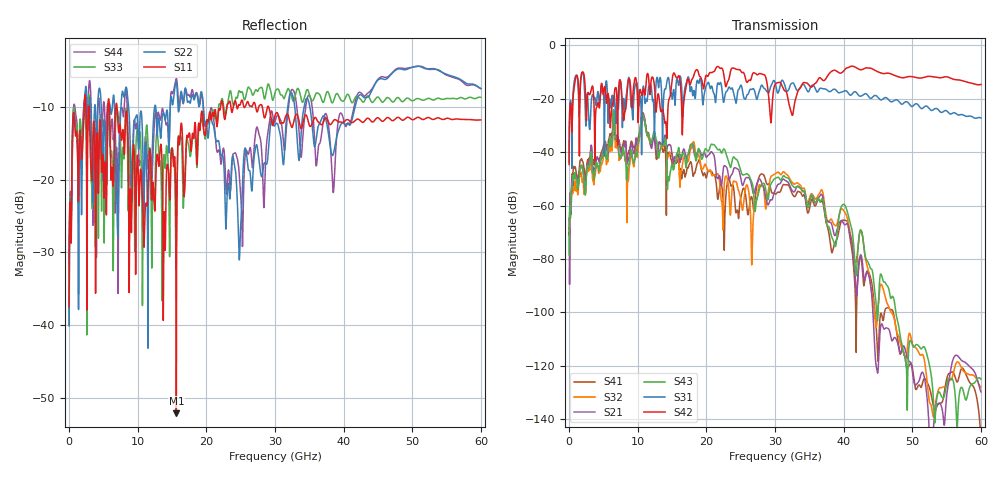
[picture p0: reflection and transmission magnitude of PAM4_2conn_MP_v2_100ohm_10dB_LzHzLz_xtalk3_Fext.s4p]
! Info: Touchstone file created by Circ.  Input file=FAB50GbE_2conn_Midplane_Examax_Topo2_v2_100ohm_10dB_LzHzLz.circ
# Hz S RI R 50
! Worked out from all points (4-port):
!   6000 points, 10 MHz to 60 GHz, reference 50 ohm
!   strongest paths, dB at 10 MHz, 15.01 GHz, 30.01 GHz, 45.01 GHz, 60 GHz:
!     S42: -44.7, -13.0, -14.7, -9.9, -14.7
!     S31: -43.6, -19.7, -13.9, -19.5, -27.2
!     S43: -78.4, -44.6, -49.9, -100.4, -125.0
!     S21: -64.7, -41.3, -54.3, -122.1, -129.7
!     S32: -69.2, -40.5, -48.2, -98.8, -128.0
!     S41: -68.5, -44.2, -55.6, -118.3, -146.4
!   lowest |S11| = -52.1 dB at 15.63 GHz (marker M1), VSWR 1.00, Z = 49.8 + j0.0187 ohm
!   |S11| at or under -10 dB: 2.897 GHz to 5.662 GHz (2.765 GHz wide, 64.6 % of centre); 6.985 GHz to 22.08 GHz (15.1 GHz wide, 104 % of centre); 29.07 GHz to end of sweep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
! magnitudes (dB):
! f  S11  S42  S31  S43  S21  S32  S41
! 10 MHz  -37.4  -44.7  -43.6  -78.4  -64.7  -69.2  -68.5
! 980 MHz  -13.9  -12.0  -11.3  -49.9  -48.8  -53.0  -46.7
! 6.61 GHz  -14.1  -17.9  -19.0  -27.0  -29.7  -30.6  -27.6
! 15.63 GHz  -52.1  -12.0  -13.6  -41.4  -41.9  -43.3  -44.1
! 24.85 GHz  -9.8  -9.1  -15.9  -45.6  -47.7  -55.6  -59.9
! 41.79 GHz  -11.8  -8.3  -17.5  -86.2  -90.7  -81.4  -104.0
! 60 GHz  -11.8  -14.7  -27.2  -125.0  -129.7  -128.0  -146.4
